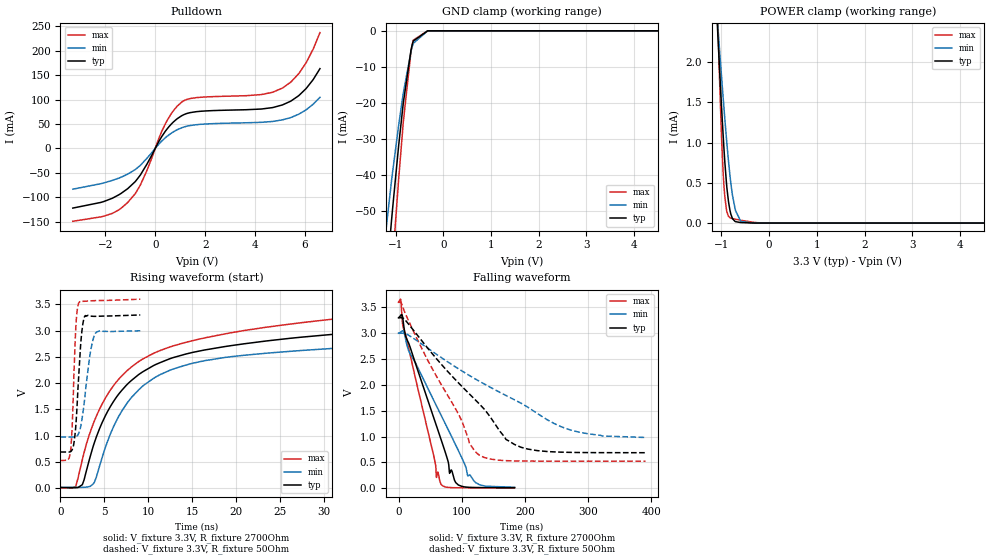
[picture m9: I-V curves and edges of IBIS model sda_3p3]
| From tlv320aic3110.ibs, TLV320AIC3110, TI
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|   sda_3p3 Model
[Model]   sda_3p3
Model_type   I/O_open_drain
Polarity   Inverting
Vinl = 0.99
Vinh = 2.31
Vmeas = 1.65
Vref = 3.3
Cref = 110pF
Rref = 2700
|   typ   min   max
|   (nom PVT)   (fast PVT)   (slow PVT)
C_comp   1.236e-12   1.219e-12   1.236e-12
[Model spec]
Vinl   0.99   0.90   1.08
Vinh   2.31   2.10   2.52
| Where nom  PVT is Nominal Process, 3.3V, 27C
|   Fast PVT is Strong Process,  3.6V, -40C
|   Slow PVT is Weak Process,   3V, 125C
[Voltage Range]   3.3   3   3.6
|Junction Temperature
[Temperature Range]   27   125   -40
[Pullup Reference]   3.3   3   3.6
[Pulldown Reference]   0   0   0
[Power Clamp Reference]   3.3   3   3.6
[GND Clamp Reference]   0   0   0
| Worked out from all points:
|   slope of the pulldown table from 0 to 0.495 V, typ, clamps not added: 12.1 ohm
|   POWER clamp passes 1 mA (typ) near -0.95 V on its own axis
|   falling waveform, V_fixture 3.3V, R_fixture 2700Ohm: 20-80 % time 54ns typ, 71.3ns min, 40.8ns max; typ from 3.3 V to 0.012 V
|   rising waveform, V_fixture 3.3V, R_fixture 2700Ohm: 20-80 % time 13.3ns typ, 10.8ns min, 14.3ns max; typ from 0.012 V to 3.3 V
|   falling waveform, V_fixture 3.3V, R_fixture 50Ohm: 20-80 % time 113ns typ, 168ns min, 79.4ns max; typ from 3.3 V to 0.689 V
|   rising waveform, V_fixture 3.3V, R_fixture 50Ohm: 20-80 % time 563ps typ, 907ps min, 397ps max; typ from 0.689 V to 3.3 V
[Pulldown]
|   Voltage   I(typ)   I(min)   I(max)
-3.3V     -122.2mA   -83.45mA   -149.3mA
-1.712V   -102mA     -65.44mA   -133mA
-1.097V   -82.21mA   -52.52mA   -110.5mA
-596.4mV  -54.58mA   -34.72mA   -75.17mA
459mV     38.8mA     24.15mA    55.49mA
1.049V    66.64mA    42.09mA    94.49mA
1.65V     75.37mA    48.67mA    104.1mA
4.256V    80.8mA     53.54mA    110.4mA
5.099V    89.22mA    58.59mA    123.8mA
5.451V    97.6mA     63.67mA    136.9mA
6.039V    122.4mA    78.96mA    175.2mA
6.6V      163.6mA    104.8mA    237.5mA
[GND Clamp]
|   Voltage   I(typ)   I(min)   I(max)
-3.3V     -1.799A    -1.559A    -1.981A
-1.47V    -113.7mA   -86.89mA   -144.9mA
-1.09V    -53.03mA   -41.95mA   -68.9mA
-1.066V   -49.56mA   -39.38mA   -64.41mA
-937.2mV  -31.82mA   -26.19mA   -41.11mA
-841.2mV  -20.14mA   -17.39mA   -25.46mA
-678mV    -5.292mA   -5.667mA   -5.59mA
-653.4mV  -3.859mA   -4.421mA   -3.807mA
-632.4mV  -2.845mA   -3.494mA   -2.609mA
-330mV    -1.164uA   -11.12uA   -122.9nA
6.6V      0A         0A         0A
[POWER Clamp]
|   Voltage   I(typ)   I(min)   I(max)
-3.3V     32.44mA    22.56mA    56.44mA
-1.096V   2.591mA    2.619mA    2.932mA
-1.043V   1.961mA    2.185mA    1.866mA
-999.6mV  1.472mA    1.84mA     1.108mA
-963.6mV  1.093mA    1.56mA     627.4uA
-927.6mV  755.3uA    1.29mA     324.1uA
-882mV    420.9uA    968.9uA    132.5uA
-822mV    162.1uA    599.1uA    66.58uA
-702.9mV  17.31uA    153.9uA    47.23uA
-594mV    6.199uA    19.71uA    34.8uA
-330mV    249.7nA    22.98nA    9.678uA
6.6V      0A         0A         0A
[Ramp]
R_load = 2700
|   typ   min   max
dV/dt_r   1.97298/1.32647e-08   1.78952/1.08894e-08   2.15442/1.42232e-08
dV/dt_f   1.97298/5.40251e-08   1.78952/7.13617e-08   2.15442/4.07629e-08
[Falling Waveform]
V_fixture = 3.3V
V_fixture_min = 3V
V_fixture_max = 3.6V
R_fixture = 2700Ohm
|   Time   V(typ)   V(min)   V(max)
0s        3.3V       3V         3.6V
3.46ns    3.346V     3.022V     3.654V
5.82ns    3.35V      3.045V     3.257V
11.06ns   2.955V     2.901V     2.986V
56.2ns    1.349V     1.691V     604.6mV
60.02ns   1.211V     1.596V     210.3mV
80.84ns   290.5mV    1.081V     15.73mV
94.74ns   63.89mV    729.6mV    10.58mV
122.3ns   15.38mV    109.3mV    9.029mV
183.7ns   11.78mV    19.89mV    8.788mV
[Rising Waveform]
V_fixture = 3.3V
V_fixture_min = 3V
V_fixture_max = 3.6V
R_fixture = 2700Ohm
|   Time   V(typ)   V(min)   V(max)
0s        11.7mV     17.46mV    8.814mV
1.74ns    9.004mV    17.01mV    32.35mV
2.5ns     70.27mV    15.63mV    550mV
3.82ns    845.4mV    100.3mV    1.262V
6.06ns    1.656V     1.176V     1.957V
8.08ns    2.051V     1.726V     2.307V
12.78ns   2.483V     2.266V     2.706V
23.44ns   2.803V     2.57V      3.065V
61.92ns   3.197V     2.871V     3.516V
161.3ns   3.299V     2.995V     3.6V
[Falling Waveform]
V_fixture = 3.3V
V_fixture_min = 3V
V_fixture_max = 3.6V
R_fixture = 50Ohm
|   Time   V(typ)   V(min)   V(max)
0s        3.3V       3V         3.6V
10.1ns    3.264V     2.996V     3.401V
46.9ns    2.702V     2.707V     2.462V
95.69ns   2.031V     2.307V     1.418V
112.3ns   1.824V     2.183V     864mV
128ns     1.633V     2.072V     642.6mV
170ns     947.2mV    1.797V     535.8mV
194.8ns   791.2mV    1.641V     528.2mV
269.7ns   696mV      1.138V     525.5mV
391.2ns   689mV      983.6mV    525.4mV
[Rising Waveform]
V_fixture = 3.3V
V_fixture_min = 3V
V_fixture_max = 3.6V
R_fixture = 50Ohm
|   Time   V(typ)   V(min)   V(max)
0s        688.8mV    973.7mV    525.4mV
1.13ns    692.6mV    973.8mV    668.8mV
1.35ns    740.1mV    973.7mV    1.228V
1.73ns    1.144V     976.7mV    3.007V
2.07ns    2.108V     1.041V     3.524V
2.34ns    2.814V     1.203V     3.557V
2.66ns    3.221V     1.562V     3.559V
3.35ns    3.276V     2.527V     3.566V
3.97ns    3.272V     2.946V     3.571V
9.089ns   3.298V     2.997V     3.599V
